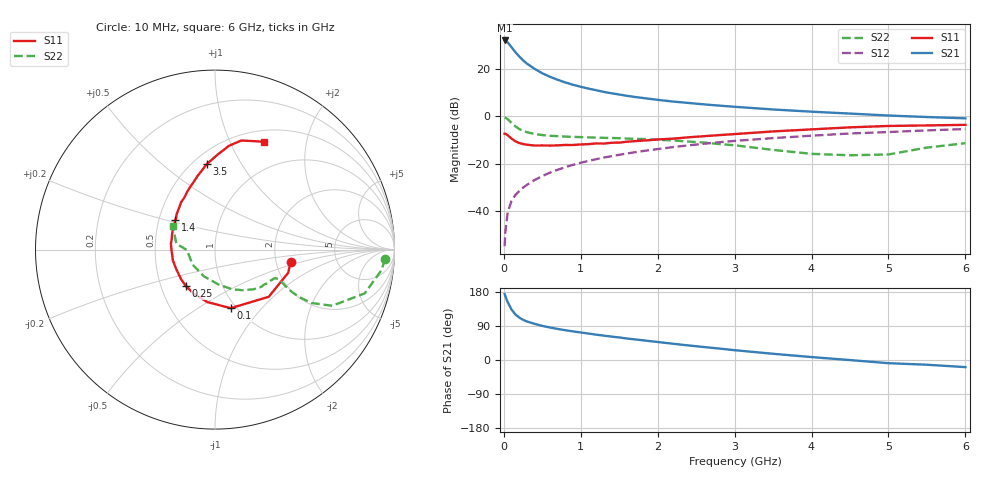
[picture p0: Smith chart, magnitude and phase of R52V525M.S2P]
! SIEMENS Small Signal Semiconductors
! BFR183
! Si NPN RF Bipolar Junction Transistor in SOT23
! VCE = 2.5 V  IC = 25 mA
! Common Emitter S-Parameters:  May  1996
# GHz  S  MA  R  50
!  f  S11  S21  S12  S22
! GHz  MAG  ANG  MAG  ANG  MAG  ANG  MAG  ANG
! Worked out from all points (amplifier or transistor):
!   36 points, 10 MHz to 6 GHz, reference 50 ohm
!   highest |S21| = 32.1 dB at 10 MHz (marker M1)
!   |S21| within 3 dB of that: start of sweep to 104 MHz
!   unconditionally stable (mu >= 1): 454.8 MHz to 2.345 GHz
!   at 250 MHz: K = 0.87, MSG = 26.9 dB, |S12| = -30.1 dB
!   at 1.4 GHz: K = 1.05, MAG = 11.9 dB, |S12| = -16.9 dB
!   at 6 GHz: K = 0.91, MSG = 2.3 dB, |S12| = -5.4 dB
!   S11 on the Smith chart (normalised r, x): 10 MHz: 2.42, -0.40; 100 MHz: 0.94, -0.70; 250 MHz: 0.67, -0.29; 1.4 GHz: 0.61, +0.21; 3.5 GHz: 0.58, +0.72; 6 GHz: 0.63, +1.35
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0.01  0.4277 -9.0  40.09 174.0  0.0018 86.6  0.9483 -3.2
0.02  0.4277 -17.6  39.44 168.2  0.0037 79.8  0.935 -7.0
0.05  0.3985 -41.3  36.41 152.6  0.0093 78.7  0.8692 -16.3
0.1  0.3379 -74.9  28.94 133.1  0.0163 72.2  0.724 -25.6
0.15  0.2957 -98.1  22.71 120.2  0.0217 69.3  0.6134 -29.0
0.2  0.2732 -115.8  18.39 112.0  0.0262 68.9  0.541 -29.4
0.25  0.2593 -129.1  15.27 106.1  0.0311 70.3  0.4917 -28.9
0.3  0.2509 -138.8  13.03 101.7  0.0356 71.0  0.4621 -28.1
0.4  0.2415 -154.3  10.05 95.4  0.045 72.0  0.4237 -26.5
0.5  0.2424 -165.6  8.118 90.0  0.0546 72.9  0.4009 -25.3
0.6  0.2405 -174.0  6.84 85.8  0.0645 72.6  0.3881 -25.0
0.7  0.2431 179.2  5.915 82.0  0.0744 72.7  0.3805 -25.2
0.8  0.248 172.1  5.193 78.6  0.0842 72.1  0.3727 -25.4
0.9  0.2478 166.5  4.64 75.5  0.0943 71.5  0.3671 -25.9
1.1  0.2579 156.3  3.853 69.8  0.1143 70.3  0.359 -28.2
1.4  0.276 143.8  3.064 61.8  0.1437 67.5  0.3486 -31.8
1.7  0.2984 134.0  2.567 54.4  0.1735 64.4  0.3344 -36.3
2.2  0.3371 120.3  2.049 42.9  0.2235 58.8  0.3089 -45.7
3.5  0.4791 95.4  1.394 16.4  0.3462 41.9  0.1948 -84.6
4.5  0.5839 82.3  1.142 -0.2  0.4338 28.9  0.1503 -146.5
5.5  0.6415 70.4  0.965 -12.5  0.5044 17.0  0.2182 171.2
6  0.6598 65.6  0.906 -18.8  0.5371 9.3  0.2702 150.4
